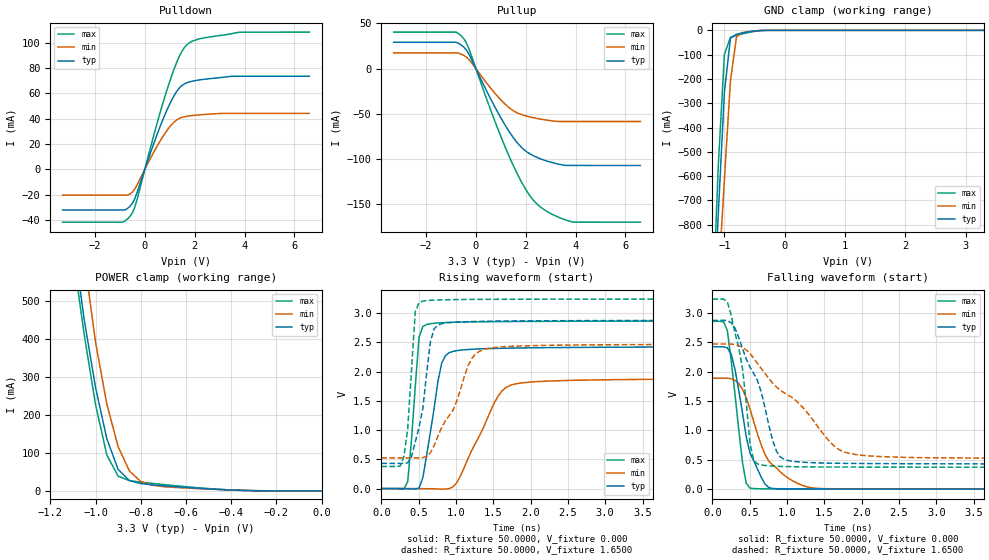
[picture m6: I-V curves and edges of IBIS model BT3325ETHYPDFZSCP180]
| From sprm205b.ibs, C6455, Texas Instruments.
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|   Model BT3325ETHYPDFZSCP180
[Model]   BT3325ETHYPDFZSCP180
Model_type   I/O
Polarity   Non-Inverting
Enable   Active-Low
Vinl =   0.8000V
Vinh =   2.0000V
Vmeas =   1.5000V
Cref =  20.0000pF
Rref =  25.0000
Vref =   1.5000V
C_comp   2.0711pF   2.0054pF   2.1518pF
[Temperature Range]   25.0000   0.1250k   -40.0000
[Pullup Reference]   3.3000V   3.0000V   3.6000V
[Pulldown Reference]   0.000V   0.000V   0.000V
[POWER Clamp Reference]   3.3000V   3.0000V   3.6000V
[GND Clamp Reference]   0.000V   0.000V   0.000V
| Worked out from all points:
|   slope of the pulldown table from 0 to 0.495 V, typ, clamps not added: 17.8 ohm
|   slope of the pullup table from 0 to 0.495 V, typ, clamps not added: 17.6 ohm
|   GND clamp passes 1 mA (typ) near -0.42 V on its own axis
|   POWER clamp passes 1 mA (typ) near -0.32 V on its own axis
|   rising waveform, R_fixture 50.0000, V_fixture 0.000: 20-80 % time 179ps typ, 414ps min, 102ps max; typ from 0 V to 2.42 V
|   rising waveform, R_fixture 50.0000, V_fixture 1.6500: 20-80 % time 166ps typ, 391ps min, 90.4ps max; typ from 0.43 V to 2.87 V
|   falling waveform, R_fixture 50.0000, V_fixture 0.000: 20-80 % time 237ps typ, 376ps min, 150ps max; typ from 2.42 V to 0 V
|   falling waveform, R_fixture 50.0000, V_fixture 1.6500: 20-80 % time 384ps typ, 865ps min, 190ps max; typ from 2.87 V to 0.429 V
[Pulldown]
| voltage   I(typ)   I(min)   I(max)
-3.3V     -32.13mA   -20.39mA   -41.8mA
-800mV    -32.13mA   NA         -40.84mA
-600mV    -29.35mA   -19.57mA   -37.3mA
-400mV    -23.06mA   -15.47mA   -29.75mA
400mV     22.69mA    15.1mA     29.91mA
900mV     47.48mA    31.04mA    63.55mA
1.2V      59.18mA    37.83mA    80.66mA
1.4V      64.67mA    40.4mA     90mA
1.7V      68.56mA    41.99mA    98.77mA
2.2V      70.71mA    43.08mA    103.2mA
3.5V      73.58mA    NA         107.3mA
6.6V      73.58mA    44.26mA    108.5mA
[Pullup]
| voltage   I(typ)   I(min)   I(max)
-3.3V     29.23mA    17.5mA     40.45mA
-800mV    29.23mA    17.5mA     40.45mA
-500mV    24.25mA    14.84mA    33.71mA
-300mV    17.07mA    10.77mA    23.36mA
700mV     -39.18mA   -25.19mA   -53.66mA
1.4V      -72.33mA   -44.64mA   -101.1mA
1.8V      -86.33mA   -50.54mA   -123.9mA
2.1V      -93.14mA   -52.96mA   -138mA
2.6V      -99.86mA   -55.89mA   -153.3mA
3V        -103.5mA   -57.58mA   -160.3mA
3.6V      -107.1mA   NA         -167.4mA
6.6V      -107.2mA   -58.47mA   -169.9mA
[GND_clamp]
| voltage   I(typ)   I(min)   I(max)
-3.3V     -15.89A    -14.36A    -17.09A
-1.2V     -1.272A    -1.463A    -1.17A
-1.1V     -747.7mA   -1.03A     -548.7mA
-1V       -253mA     -613mA     -98.95mA
-900mV    -32.84mA   -207.1mA   -28.45mA
-800mV    -15.85mA   -27.49mA   -20.55mA
-700mV    -10.61mA   -9.139mA   -14.42mA
-400mV    -643.6uA   -604.1uA   -1.057mA
3.3V      40.31nA    12.94uA    313.1nA
[POWER_clamp]
| voltage   I(typ)   I(min)   I(max)
-3.3V     13.85A     12.5A      14.97A
-1.1V     674.6mA    860.3mA    626.3mA
-1.05V    451.8mA    613.5mA    412.5mA
-1V       273.4mA    392.8mA    228.3mA
-950mV    137.5mA    229mA      94.82mA
-900mV    56.64mA    116.9mA    38.99mA
-850mV    27.27mA    52.59mA    27.18mA
-800mV    19.38mA    24.87mA    23.13mA
-750mV    16.1mA     15.12mA    19.91mA
-600mV    9.256mA    7.601mA    11.11mA
-350mV    1.398mA    1.65mA     1.22mA
0V        527.1nA    2.815uA    493.3nA
[Ramp]
| variable   typ   min   max
dV/dt_r   1.4534/0.1776n   1.1263/0.4102n   1.7179/0.1008n
dV/dt_f   1.4432/0.2658n   1.1309/0.5695n   1.6967/0.1542n
R_load = 50.0000
[Rising Waveform]
R_fixture = 50.0000
V_fixture = 0.000
V_fixture_min = 0.000
V_fixture_max = 0.000
| time   V(typ)   V(min)   V(max)
0s        36.98uV    40.38uV    55.68uV
353.5ps   -4.286mV   51.88uV    118.7mV
404ps     -5.188mV   53.98uV    828mV
505.1ps   8.002mV    -314.8uV   2.581V
606.1ps   556.7mV    -3.177mV   2.804V
808.1ps   2.14V      -9.65mV    2.834V
959.6ps   2.344V     27.59mV    2.842V
1.515ns   2.394V     1.467V     2.853V
1.717ns   2.4V       1.759V     2.854V
5ns       2.422V     1.877V     2.863V
[Rising Waveform]
R_fixture = 50.0000
V_fixture = 1.6500
V_fixture_min = 1.5000
V_fixture_max = 1.8000
| time   V(typ)   V(min)   V(max)
0s        429.6mV    524.6mV    377.1mV
303ps     429.2mV    524.8mV    549.8mV
353.5ps   441.4mV    524.8mV    1.016V
454.5ps   794.9mV    524.7mV    3.021V
505.1ps   1.046V     524.7mV    3.176V
656.6ps   2.506V     608.6mV    3.217V
808.1ps   2.817V     1.041V     3.225V
1.212ns   2.854V     2.221V     3.232V
1.414ns   2.859V     2.39V      3.233V
5ns       2.874V     2.466V     3.238V
[Falling Waveform]
R_fixture = 50.0000
V_fixture = 0.000
V_fixture_min = 0.000
V_fixture_max = 0.000
| time   V(typ)   V(min)   V(max)
0s        2.424V     1.889V     2.858V
151.5ps   2.425V     1.889V     2.85V
202ps     2.402V     1.889V     2.695V
303ps     2.043V     1.853V     1.618V
404ps     1.298V     1.701V     449.6mV
454.5ps   885.8mV    1.552V     98.1mV
505.1ps   611.6mV    1.362V     19.06mV
757.6ps   27.94mV    475.9mV    4.505mV
1.263ns   4.632mV    41.03mV    1.261mV
5ns       244.9uV    1.426mV    23.63uV
[Falling Waveform]
R_fixture = 50.0000
V_fixture = 1.6500
V_fixture_min = 1.5000
V_fixture_max = 1.8000
| time   V(typ)   V(min)   V(max)
0s        2.874V     2.472V     3.236V
202ps     2.869V     2.473V     3.181V
252.5ps   2.832V     2.47V      2.958V
404ps     2.395V     2.412V     2.054V
505.1ps   2.076V     2.31V      770.4mV
606.1ps   1.845V     2.139V     428.8mV
858.6ps   647.5mV    1.739V     390.1mV
1.01ns    489.3mV    1.606V     384.5mV
1.818ns   438.9mV    614.2mV    376.7mV
5ns       428.8mV    524.5mV    374.2mV
